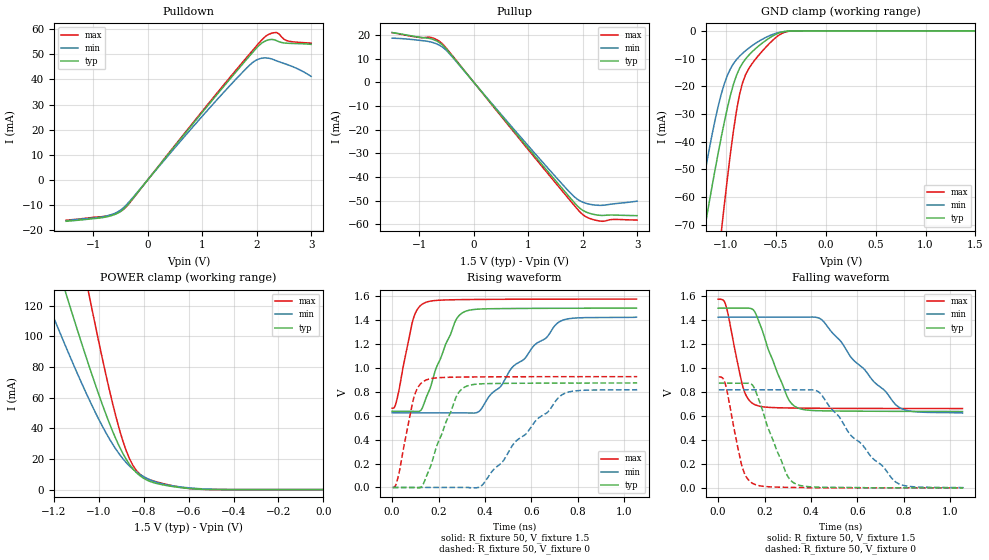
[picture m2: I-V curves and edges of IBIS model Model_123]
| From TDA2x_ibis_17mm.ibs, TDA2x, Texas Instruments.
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| Model based on original model for DDR_SEIOPB_V
|   Sub model SR010_DRV34_1P5
[model]   Model_123
|[Description]  [1.5V-I/O-X-X]
|   , ,
|[Input Load]
|[Output Drive]
|Voltage   1.5V
|Mode   I/O
Model_type   I/O
Polarity   Non-Inverting
Enable   Active-Low
Vinl =  0.65
Vinh =  0.85
Cref =  15.0000pF
Rref =  100.0000M
Vref =  0V
Vmeas =  0.75
C_comp   2p   2p   2p
[Model Spec]
Vinl   0.65   0.6125   0.6875
Vinh   0.85   0.8125   0.8875
[Receiver Thresholds]
Tslew_ac = 0.5n
Vth= 0.75
Vth_max= 0.7875
Vth_min= 0.675
Vinh_ac= 0.175
Vinh_dc= 0.1
Vinl_ac= -0.175
Vinl_dc= -0.1
[Temperature Range]   25   125   -40
[Voltage Range]   1.5   1.425   1.575
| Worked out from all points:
|   slope of the pulldown table from 0 to 0.225 V, typ, clamps not added: 36.8 ohm
|   slope of the pullup table from 0 to 0.225 V, typ, clamps not added: 35.8 ohm
|   GND clamp passes 1 mA (typ) near -0.48 V on its own axis
|   POWER clamp passes 1 mA (typ) near -0.62 V on its own axis
|   rising waveform, R_fixture 50, V_fixture 1.5: 20-80 % time 100ps typ, 242ps min, 55.8ps max; typ from 0.637 V to 1.5 V
|   rising waveform, R_fixture 50, V_fixture 0: 20-80 % time 99.3ps typ, 236ps min, 56ps max; typ from 0 V to 0.874 V
|   falling waveform, R_fixture 50, V_fixture 1.5: 20-80 % time 99.7ps typ, 222ps min, 57.6ps max; typ from 1.5 V to 0.637 V
|   falling waveform, R_fixture 50, V_fixture 0: 20-80 % time 99.9ps typ, 227ps min, 57.1ps max; typ from 0.874 V to 0 V
[POWER_clamp]
-1.5V     302.8mA    223.9mA    484.4mA
-1.242V   174.3mA    127.3mA    279.1mA
-1.136V   123.3mA    89.68mA    196.8mA
-1.045V   81.65mA    59.62mA    128.8mA
-1.03V    75mA       54.92mA    117.8mA
-939.4mV  38.44mA    29.91mA    56.84mA
-893.9mV  23.93mA    20.41mA    32.31mA
-848.5mV  13.61mA    13.43mA    15.91mA
-803mV    7.623mA    8.663mA    8.564mA
-712.1mV  3.022mA    3.561mA    3.877mA
-575.8mV  470.5uA    872uA      449uA
0V        112.6nA    435.6nA    613.8nA
[Pulldown]
-1.5V     -16.54mA   -16.32mA   -16.11mA
-727.3mV  -14.62mA   -14.26mA   -14.29mA
-545.5mV  -13.24mA   -12.72mA   -13.05mA
-409.1mV  -10.94mA   -10.36mA   -11.07mA
1.227V    32.84mA    30.87mA    33.41mA
1.818V    48.09mA    44.61mA    48.84mA
2V        52.62mA    47.82mA    53.46mA
2.182V    55.55mA    48.58mA    57.5mA
2.273V    55.99mA    48.2mA     58.42mA
2.364V    55.5mA     47.46mA    58.71mA
2.545V    54.48mA    46.06mA    55.55mA
3V        54mA       41.23mA    54.49mA
[Pullup]
-1.5V     20.96mA    18.6mA     20.95mA
-1V       19mA       17.69mA    18.93mA
-772.7mV  18.26mA    16.89mA    18.84mA
-590.9mV  16.04mA    15.07mA    16.54mA
-409.1mV  11.43mA    11.07mA    11.7mA
1.409V    -38.97mA   -37.46mA   -39.88mA
1.773V    -48.83mA   -46.66mA   -49.96mA
1.909V    -52.33mA   -49.44mA   -53.68mA
2.045V    -54.57mA   -50.97mA   -56.55mA
2.273V    -56.03mA   -51.89mA   -58.38mA
2.591V    -56.03mA   -51.23mA   -57.86mA
3V        -56.26mA   -50.14mA   -58.12mA
[GND_clamp]
-1.5V     -133.6mA   -115.7mA   -234.3mA
-1.288V   -87.29mA   -67.59mA   -156.8mA
-1.197V   -68.11mA   -48.64mA   -124.4mA
-1.045V   -38.25mA   -22.77mA   -72.51mA
-1.015V   -32.88mA   -19.1mA    -62.74mA
-954.5mV  -23.3mA    -13.72mA   -44.4mA
-863.6mV  -13.6mA    -9.192mA   -23.11mA
-803mV    -10.18mA   -7.193mA   -15.89mA
-681.8mV  -5.771mA   -4.027mA   -9.287mA
-500mV    -1.264mA   -914.7uA   -2.429mA
-348.5mV  -52.39uA   -75.11uA   -85.87uA
1.5V      112.6nA    528.1nA    514.5nA
[Ramp]
dV/dt_f 0.51818867/99.763667p 0.48136236/0.22283151n 0.54803399/57.607376p
dV/dt_r 0.52646955/99.76841p  0.49342891/0.23750758n 0.55793354/56.100375p
R_load = 50
[Rising Waveform]
R_fixture = 50
V_fixture = 1.5
V_fixture_min = 1.425
V_fixture_max = 1.575
0s        637.3mV    624.3mV    663.1mV
21.04ps   636.8mV    624.2mV    738.2mV
92.12ps   636.3mV    624.2mV    1.416V
140.2ps   717.7mV    624.2mV    1.544V
270.3ps   1.382V     624.1mV    1.57V
313.2ps   1.471V     623.1mV    1.571V
376.7ps   1.492V     639.5mV    1.573V
516.9ps   1.497V     1.003V     1.574V
721.7ps   1.499V     1.387V     1.575V
1.053ns   1.5V       1.425V     1.575V
[Rising Waveform]
R_fixture = 50
V_fixture = 0
V_fixture_min = 0
V_fixture_max = 0
2.954ps   0V         0V         0V
27.64ps   0V         0V         102.4mV
95.61ps   0V         0V         764.4mV
144.2ps   74.87mV    0V         896.6mV
274.4ps   749.8mV    0V         922.5mV
317.8ps   844.3mV    0V         923.7mV
386.8ps   866.9mV    16.92mV    924.8mV
528ps     871.2mV    375.6mV    926mV
735.3ps   872.9mV    778.8mV    926.5mV
1.056ns   874.1mV    819mV      926.7mV
[Falling Waveform]
R_fixture = 50
V_fixture = 1.5
V_fixture_min = 1.425
V_fixture_max = 1.575
0s        1.5V       1.425V     1.575V
35.09ps   1.5V       1.425V     1.511V
112.1ps   1.5V       1.425V     809.3mV
160.6ps   1.46V      1.425V     692.6mV
296.2ps   766.9mV    1.425V     667.1mV
340.4ps   669.7mV    1.425V     665.9mV
447.6ps   643.1mV    1.401V     664.1mV
579.1ps   640.3mV    1.074V     663mV
781.6ps   638.6mV    670.1mV    662.5mV
1.053ns   637.3mV    624.3mV    662.3mV
[Falling Waveform]
R_fixture = 50
V_fixture = 0
V_fixture_min = 0
V_fixture_max = 0
2.954ps   874.1mV    819mV      926.7mV
32.39ps   874.3mV    819.1mV    857.4mV
106.9ps   873.9mV    819.1mV    154.5mV
154.7ps   838.3mV    819.1mV    31.55mV
291.9ps   126.8mV    819mV      4.347mV
334.5ps   32.42mV    818.8mV    3.031mV
437.3ps   5.854mV    794.2mV    0V
569.4ps   2.773mV    443.8mV    0V
770.1ps   0V         42.46mV    0V
1.056ns   0V         0V         0V
